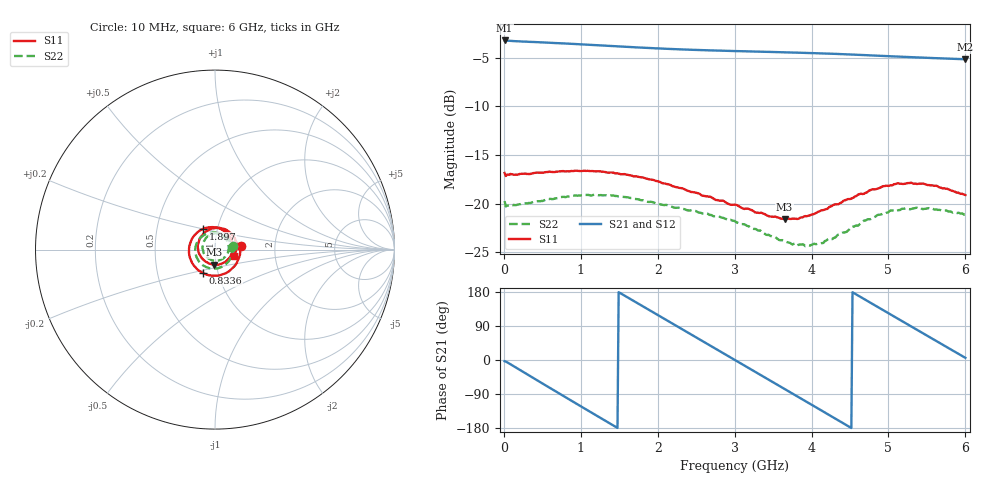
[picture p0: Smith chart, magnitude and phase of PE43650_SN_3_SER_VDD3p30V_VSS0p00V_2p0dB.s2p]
!Keysight Technologies,N5245B,MY57181451,A.13.50.07
!Date: Tuesday, May 07, 2019 07:59:48
!Correction: S11(Full 2 Port(1,2))
!S21(Full 2 Port(1,2))
!S12(Full 2 Port(1,2))
!S22(Full 2 Port(1,2))
!S2P File: Measurements: S11, S21, S12, S22:
# Hz S  dB  R 50
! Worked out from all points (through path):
!   401 points, 10 MHz to 6 GHz, reference 50 ohm
!   highest |S21| = -3.24 dB at 10 MHz (marker M1); lowest = -5.2 dB at 6 GHz (marker M2)
!   group delay of S21, straight-line fit = 330 ps
!   lowest |S11| = -21.6 dB at 3.649 GHz (marker M3), VSWR 1.18, Z = 48.7 - j8.16 ohm
!   |S11| at or under -10 dB: start of sweep to end of sweep
!   |S22| runs from -24.4 to -19.1 dB; largest |S21 - S12| = 0.0048
!   S11 on the Smith chart (normalised r, x): 10 MHz: 1.33, +0.05; 833.6 MHz: 0.85, -0.23; 1.897 GHz: 0.85, +0.20; 6 GHz: 1.23, -0.09
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1e7  -16.84 7.2  -3.24 -3.2  -3.28 -3.2  -19.73 12.8
2.34625e8  -16.93 -34.3  -3.35 -29.4  -3.39 -29.4  -19.99 -34.5
4.74225e8  -16.82 -68.2  -3.43 -58.6  -3.48 -58.6  -19.75 -68.6
8.33625e8  -16.67 -116.5  -3.57 -102.1  -3.62 -102.1  -19.25 -116.4
1.013325e9  -16.64 -139.5  -3.65 -123.7  -3.70 -123.7  -19.11 -138.3
1.4476e9  -16.88 169.1  -3.83 -175.7  -3.89 -175.6  -19.21 173.7
1.89685e9  -17.50 119.9  -4.01 131.0  -4.08 131.0  -19.82 129.5
2.01665e9  -17.74 107.4  -4.06 116.8  -4.11 116.8  -20.00 118.4
2.241275e9  -18.31 83.8  -4.14 90.2  -4.19 90.3  -20.42 97.8
2.4659e9  -18.82 59.7  -4.20 63.7  -4.26 63.7  -20.71 76.8
2.750425e9  -19.61 28.9  -4.28 30.1  -4.33 30.2  -21.29 48.9
3.005e9  -20.10 -2.2  -4.32 0.0  -4.38 0.1  -21.80 21.5
3.3045e9  -20.93 -42.5  -4.39 -35.4  -4.44 -35.4  -22.75 -16.2
3.648925e9  -21.57 -94.4  -4.46 -76.3  -4.50 -76.2  -23.84 -66.9
4.008325e9  -21.11 -152.0  -4.54 -118.9  -4.59 -118.9  -24.19 -127.4
4.2629e9  -20.24 169.3  -4.61 -149.2  -4.66 -149.1  -23.65 -169.8
4.5025e9  -19.51 136.0  -4.68 -177.7  -4.73 -177.5  -22.56 153.3
4.7421e9  -18.69 105.0  -4.76 153.9  -4.82 154.0  -21.59 121.9
5.01165e9  -18.15 73.7  -4.86 122.1  -4.91 122.2  -20.77 89.7
5.4609e9  -17.96 26.9  -5.01 69.1  -5.05 69.2  -20.53 45.3
5.745425e9  -18.46 1.4  -5.10 35.6  -5.14 35.7  -20.69 21.6
6e9  -19.11 -18.8  -5.17 5.7  -5.22 5.8  -21.14 4.6
